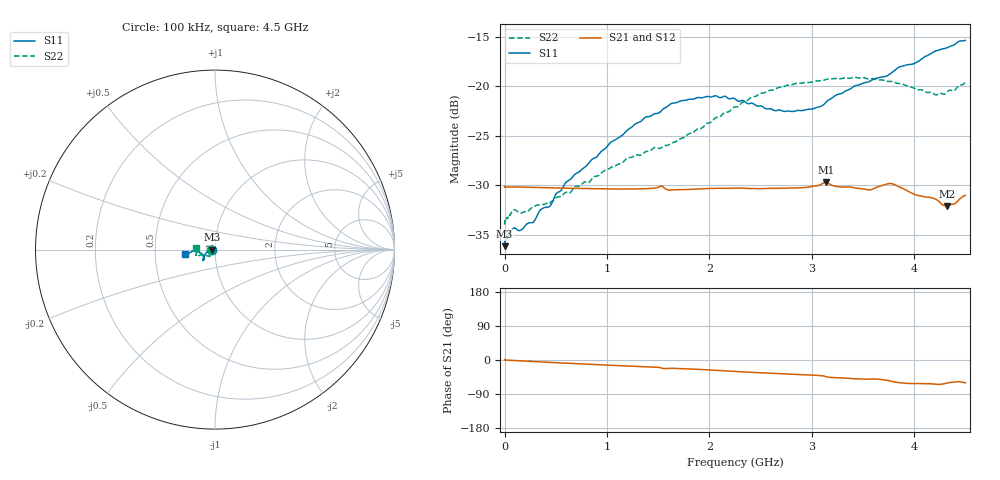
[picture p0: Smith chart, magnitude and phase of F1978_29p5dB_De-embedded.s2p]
! Integrated Device Technology
! Corporate Headquarters
! 6024 Silver Creek Valley Road
! San Jose, CA 95138  USA
! Phone:  1-408-284-8200
! Toll Free:  1-800-223-1366
! Webpage:  http://www.idt.com/
! Timing and RF Division
! 515 Groton Road, Suite 102
! Westford, MA 01886-6024
! Device:  F1978
! Description: 6-bit, 75 ohm, 0.5 dB Digital Step Attenuator
! Frequency:  5.0 MHz -  3.00 GHz
! Package:  4x4 mm QFN Plastic Package: 20 pin
! Ports:  2 RF, 11 DC
!  Pin  1  = D5 (16 dB)
!  Pin  2  = RF1  =  Port 1
!  Pin  3  = Serial Data In (DATA)
!  Pin  4  = Serial Clock (CLK)
!  Pin  5  = Serial Latch Enable (LE)
!  Pin  6  = VDD
!  Pin  7  = NC
!  Pin  8  = NC
!  Pin  9  = NC
!  Pin 10  = GND
!  Pin 11  = GND
!  Pin 12  = NC
!  Pin 13  = VMODE
!  Pin 14  = RF2  =  Port 2
!  Pin 15  = D4 (8 dB)
!  Pin 16  = D3 (4 dB)
!  Pin 17  = D2 (2 dB)
!  Pin 18  = NC
!  Pin 19  = D1 (1 dB)
!  Pin 20  = D0 (0.5 dB)
! State:  59
! Atten State:  29.5 dB
! Voltage:  +3.30 Volts
! Current:  0.559 mA
! Data:  The device was measured on a F1975 evaluation board which has
!  individual transmission lines to the RF pins.  Data was collected
!  using a calibrated network analyzer.  The evaluation board was
!  de-embedded using Automatic Fixture Removal (AFR).
!  The reference plane is the edge of the package pin.
! Misc:
!  Action Tracker AT0416
! Date Measured:  2018-02-08
! Date:  2018-03-26  MJV
! Note:
!  Integrated Device Technology supplies this data as a sample of measured
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# GHz S dB R 75
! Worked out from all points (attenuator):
!   291 points, 100 kHz to 4.5 GHz, reference 75 ohm
!   highest |S21| = -29.68 dB at 3.14 GHz (marker M1); lowest = -32.1 dB at 4.32 GHz (marker M2)
!   lowest |S11| = -36.1 dB at 100 kHz (marker M3), VSWR 1.03, Z = 72.7 - j0.00976 ohm
!   |S11| at or under -10 dB: start of sweep to end of sweep
!   |S22| runs from -33.9 to -19.1 dB; largest |S21 - S12| = 0.00014
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0.0001  -36.13 -179.8  -30.12 1.1  -30.12 1.2  -33.87 -179.1
0.007  -35.56 -178.5  -30.15 0.2  -30.15 0.0  -33.48 -177.4
0.08  -34.36 -176.3  -30.16 -1.2  -30.15 -1.2  -32.50 -169.7
0.16  -34.50 -177.8  -30.17 -2.4  -30.17 -2.4  -32.80 -160.0
0.28  -33.74 179.2  -30.20 -4.1  -30.20 -4.2  -32.15 -151.8
0.36  -32.37 179.5  -30.22 -5.2  -30.22 -5.2  -31.90 -144.3
0.44  -32.13 -180.0  -30.24 -6.3  -30.24 -6.3  -31.81 -138.6
0.6  -29.66 -176.6  -30.28 -8.4  -30.28 -8.4  -30.69 -132.8
0.76  -28.34 -170.0  -30.31 -10.5  -30.31 -10.5  -29.81 -128.7
1.28  -23.78 -153.2  -30.36 -16.8  -30.35 -16.7  -26.92 -124.5
1.52  -22.60 -145.0  -30.09 -20.1  -30.09 -20.1  -26.27 -131.1
1.62  -21.79 -143.2  -30.49 -22.1  -30.48 -22.1  -25.82 -134.5
1.88  -21.16 -139.1  -30.36 -24.6  -30.36 -24.5  -24.32 -147.2
2.26  -21.35 -137.8  -30.28 -30.1  -30.27 -30.2  -22.08 -157.9
2.64  -22.47 -147.3  -30.29 -35.4  -30.29 -35.4  -20.32 -159.4
3.02  -22.26 -163.7  -30.07 -40.2  -30.07 -40.3  -19.54 -160.0
3.14  -21.59 -166.5  -29.68 -44.1  -29.68 -44.1  -19.31 -160.5
3.56  -19.54 -177.0  -30.45 -50.5  -30.45 -50.5  -19.29 -165.9
3.76  -18.79 -175.7  -29.81 -55.0  -29.80 -55.0  -19.52 -169.5
4.2  -16.49 -172.5  -31.35 -63.6  -31.35 -63.6  -20.84 179.0
4.32  -16.13 -172.1  -32.07 -60.7  -32.06 -60.8  -20.64 176.6
4.5  -15.39 -171.9  -31.01 -60.2  -31.01 -60.2  -19.57 174.0
